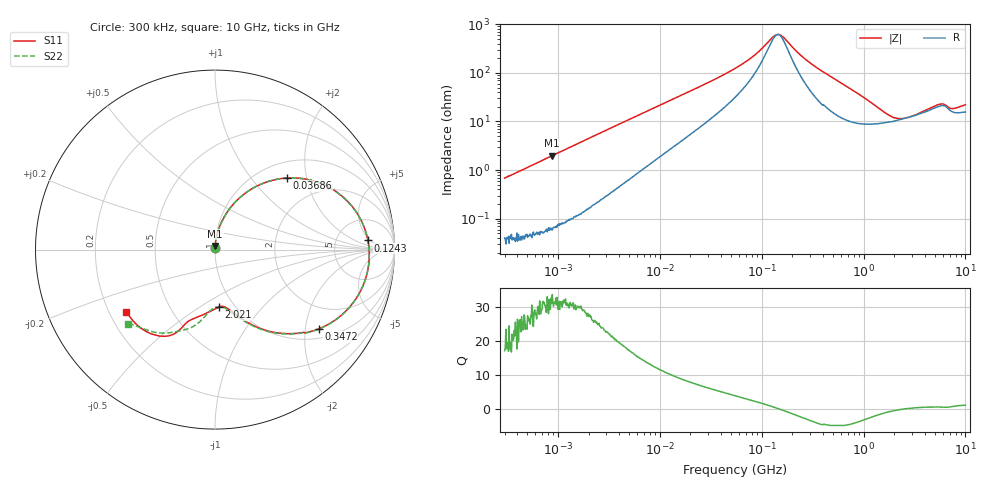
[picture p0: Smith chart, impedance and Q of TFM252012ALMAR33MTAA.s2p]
! S-Parameter Data Generated by TDK Corporation
! Copyright(C) 2019 TDK Corporation.
! All Rights Reserved.
! TDK P/N: TFM252012ALMAR33MTAA (Inductor)
! Property: L=330nH at 1MHz
! Size(LxWxT): 2.5x2x1.2mm
! Model Type: s2p (Touchstone File Format Version 1.0)
! Frequency: DC=Yes Start=0.3MHz Stop=10000MHz 802points Log-sweep
! Model Generated on May 10, 2019
! Port Assignments:
!  1 ---@@@--- 2
! Applicable Conditions:
!  Temperature = 25 degC
!  DC Bias Current = 0 A
!  Small Signal Operation
! Terms and conditions regarding TDK Simulation Models
! (1)This simulation model is being provided solely for informational purposes. Please refer to the specifications of the products in terms of detailed characteristics of such products.
! (2)In no event shall TDK Corporation of any of its subsidiaries be liable for any loss or damage arising, directly or indirectly,
!  From any information contained in this simulation model, including, but not limited to loss or damages arising from any inaccuracies, omissions or errors in connection with such information.
! (3)Any and all copyrights on this simulation model are owned by TDK Corporation.
!  Duplication or redistribution of this simulation model without prior written permission from TDK Corporation is prohibited.
! (4)This simulation model is subject to any modification or change without any prior notice.
! (5)Neither TDK Corporation nor any of its subsidiaries shall make any warranty, express or implied,
!  Including but not limited to the correctness, implied warranties of merchantability and fitness for a particular purpose with respect to this simulation models.
! (6)The use of this simulation model shall be deemed to have consented to the terms and conditions hereof.
# Hz S MA R 50
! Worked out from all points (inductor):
!   801 points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, 300 kHz to 10 GHz, reference 50 ohm
!   read as one part in series: L = 360 nH near 318.3 kHz
!   highest Q = 32.6 at 881.6 kHz (marker M1), where L = 357 nH
!   self-resonance near 144.2 MHz
!   S11 on the Smith chart (normalised r, x): 300 kHz: 1.00, +0.01; 36.86 MHz: 1.31, +1.54; 124.3 MHz: 11, +4; 347.2 MHz: 1.26, -2.36; 2.021 GHz: 0.85, -0.61; 10 GHz: 0.27, -0.30
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300000  0.006759 86.5  0.9996 -0.4  0.9992 -0.4  0.007175 88.9
881608  0.01964 87.0  0.9993 -1.1  0.9991 -1.1  0.01979 87.4
1713600  0.03806 85.8  0.998 -2.2  0.9979 -2.2  0.03817 85.8
9671944  0.2 73.4  0.9628 -11.6  0.9628 -11.6  0.2 73.4
1.945436e7  0.3632 61.3  0.8868 -21.4  0.8868 -21.4  0.3631 61.3
3.686242e7  0.5662 44.8  0.7245 -34.3  0.7244 -34.3  0.5661 44.8
5.477226e7  0.6922 32.3  0.5661 -42.9  0.5661 -42.9  0.6921 32.3
8.505279e7  0.8023 17.3  0.3498 -48.1  0.3499 -48.1  0.8022 17.2
1.242712e8  0.8538 3.4  0.1694 -29.7  0.1694 -29.7  0.8537 3.3
1.405283e8  0.8598 -1.2  0.141 -7.7  0.141 -7.7  0.8597 -1.3
1.540638e8  0.8607 -4.8  0.1448 12.1  0.1448 12.1  0.8605 -4.9
2.320257e8  0.8247 -21.0  0.327 45.6  0.327 45.6  0.8244 -21.2
3.126428e8  0.7577 -33.2  0.4916 42.3  0.4916 42.3  0.7573 -33.5
3.471693e8  0.7268 -37.5  0.5457 39.7  0.5457 39.7  0.7265 -37.7
5.105874e8  0.5927 -51.9  0.7063 27.9  0.7063 27.8  0.5926 -52.2
8.070667e8  0.4398 -66.4  0.8213 13.2  0.8213 13.2  0.4402 -66.9
1.767019e9  0.3176 -84.0  0.8603 -10.6  0.8604 -10.6  0.3195 -85.8
2.020878e9  0.3221 -86.1  0.8538 -14.7  0.8537 -14.7  0.3211 -89.7
4.632637e9  0.4326 -111.0  0.725 -43.8  0.7249 -43.9  0.4589 -107.6
6.656819e9  0.5626 -120.9  0.6217 -56.9  0.6216 -56.9  0.568 -125.7
8.09931e9  0.6032 -135.0  0.5919 -67.9  0.5918 -67.9  0.6187 -137.2
1e10  0.6039 -144.8  0.5502 -79.2  0.5503 -79.3  0.6382 -139.7
